PROGRAM MAIN
VAR 
	fbCSV: FB_CSV;
	
	{ attribute 'TcEncoding' := 'UTF-8'}
	sTemp: STRING; 
END_VAR

VAR CONSTANT
	ci_DecimalPlaces: USINT:= 3; (*保留有效数字 *)
END_VAR

IF fbCSV.bRingBufferFull THEN
	RETURN;
END_IF


iData1 := iData1 + 0.001;
iData2 := iData2 + 1;
iData3 := 'Test';
iData4 := "倍福中国";
 
Wstring_to_UTF8(ADR(sTemp), ADR(iData4),SIZEOF(iData4));


fbCSV.pRowData[1] := LREAL_TO_FMTSTR(iData1, ci_DecimalPlaces, TRUE); 
fbCSV.pRowData[2] :=INT_TO_STRING(iData2); 
fbCSV.pRowData[3] := iData3;
fbCSV.pRowData[4] := sTemp;


fbCSV(sPath:= 'D:');

END_PROGRAM
